PROGRAM MAIN
VAR
	udiCounterTemp						:UDINT;
	fbTimer								:TON;
	fbReadTaskExceedCounter				:FB_ReadTaskExceedCounter;
	
	fbTrig								:R_TRIG;
	i,iCount							:DINT;
END_VAR

fbTrig(); fbTrig.CLK;
IF fbTrig.Q THEN
	fbTrig.CLK := FALSE;
	FOR i:=1 TO 500000 BY 1 DO
		iCount := iCount * i;
	END_FOR
END_IF

Act_DetectExceedCounter();

ACTION Act_DetectExceedCounter:
fbTimer(IN:=NOT fbTimer.Q, PT:=T#100MS);

fbReadTaskExceedCounter(
    bExecute        := NOT fbReadTaskExceedCounter.bBusy AND fbTimer.Q,
    nTaskAdsPort    := _TaskInfo[GETCURTASKINDEXEX()].AdsPort,
    bBusy           => ,
    bError          => ,
    nErrorID        => ,
    nExceedCounter  => );
	
IF fbReadTaskExceedCounter.nExceedCounter <> 0
	AND_THEN udiCounterTemp <> fbReadTaskExceedCounter.nExceedCounter THEN
	udiCounterTemp := fbReadTaskExceedCounter.nExceedCounter;
	ADSLOGDINT(
        msgCtrlMask  := ADSLOG_MSGTYPE_HINT OR ADSLOG_MSGTYPE_LOG,
        msgFmtStr    := CONCAT(_TaskInfo[GETCURTASKINDEXEX()].TaskName, ' Error! Exceed counter is not zero! Current Count:%d'),
        dintArg      := udiCounterTemp);
END_IF
END_ACTION

END_PROGRAM
